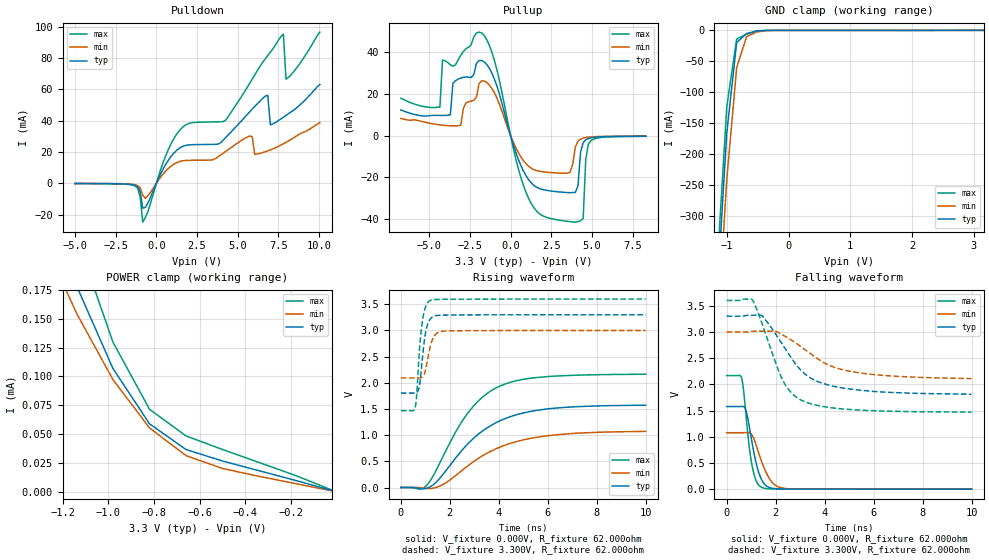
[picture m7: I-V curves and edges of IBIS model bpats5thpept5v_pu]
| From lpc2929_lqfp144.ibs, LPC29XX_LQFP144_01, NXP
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| |   Rev 0.20 IBIS Model Design Automation Generation   |
| |   N O N - S I L I C O N   C O R R E L A T E D   |
| |   This IBIS [Model] is pre-Beta tactical support   |
| |  Note: this IBIS [Model] contains clamp curves generated   |
| |   through simulation which should not be relied upon   |
| Pccmos14 hliolib_nlm 4.0.1
|   0.18 um 3.3V pad library
|   six level metal
|   dual oxide
|   single threshold voltage
|   nominal line mixed supply
|   parasitic extracted netlists
| Process block c14
| bpats5thpept5v
|   Bidirectional Pad 3v3
|   3state Output
|   Plain Input
|   5ns Slew Rate control
|   CMOS
|   Programmable between
|   - (p1=0, p2=1) plain input
|   - (p1=0, p2=0) with Pull Up
|   - (p1=1, p2=1) with Pull Down
|   - (p1=1, p2=0) with Repeater
|   Characterized at Core 1.8V and I/O 3.3V
| Pull Up Mode (p1=0, p2=0)
[Model]   bpats5thpept5v_pu | of bpats5thpept5v
Model_type   I/O
Polarity   Non-Inverting
Enable   Active-Low
|  Reciever Thresholds
Vinl   = 0.99V
Vinh   = 2.31V
| AC Test Load Conditions
Vref   = 0
Cref   = 1.2e-11
Rref   = 1000000000
Vmeas   = 1.65
| [Process Range]   typical   min   max
| C_comp edge width   400.000ps   400.000ps   400.000ps
| C_comp Tstrobe   40.000fs   40.000fs   40.000fs
C_comp   2.536pF   2.398pF   2.677pF
[Temperature Range]   25   125   -40
[Voltage Range]   3.30V   3.00V   3.60V
[GND Clamp Reference]   0.00V   0.00V   0.00V
[Pulldown Reference]   0.00V   0.00V   0.00V
[POWER Clamp Reference]   3.30V   3.00V   3.60V
[Pullup Reference]   3.30V   3.00V   3.60V
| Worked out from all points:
|   slope of the pulldown table from 0 to 0.495 V, typ, clamps not added: 46.5 ohm
|   slope of the pullup table from 0 to 0.495 V, typ, clamps not added: 41.9 ohm
|   GND clamp passes 1 mA (typ) near -0.48 V on its own axis
|   POWER clamp passes 1 mA (typ) near -2.29 V on its own axis
|   rising waveform, V_fixture 0.000V, R_fixture 62.000ohm: 20-80 % time 2.14ns typ, 2.37ns min, 1.8ns max; typ from 0.001 V to 1.57 V
|   falling waveform, V_fixture 0.000V, R_fixture 62.000ohm: 20-80 % time 411ps typ, 539ps min, 320ps max; typ from 1.58 V to 0.001 V
|   rising waveform, V_fixture 3.300V, R_fixture 62.000ohm: 20-80 % time 224ps typ, 260ps min, 214ps max; typ from 1.8 V to 3.3 V
|   falling waveform, V_fixture 3.300V, R_fixture 62.000ohm: 20-80 % time 1.53ns typ, 1.95ns min, 1.1ns max; typ from 3.3 V to 1.81 V
[GND Clamp]
| ref voltage   0.00V   0.00V   0.00V
|   Voltage   I(typ)   I(min)   I(max)
-5V       -7.933A    -7.953A    -7.929A
-1.16V    -429.6mA   -501mA     -389.4mA
-1V       -166.1mA   -240.8mA   -123.1mA
-840mV    -19.83mA   -60.19mA   -14.19mA
-680mV    -5.242mA   -10.3mA    -6.178mA
-520mV    -1.331mA   -2.714mA   -864.2uA
-200mV    -50.25uA   -41.81uA   -77.56uA
3.16V     -7.353uA   6.327uA    -29.63uA
[Power Clamp]   | Vtable = Vcc - Vpad
| ref voltage   3.30V   3.00V   3.60V
|   Voltage   I(typ)   I(min)   I(max)
-6.74V    8.239mA    4.142mA    14.64mA
-1.3V     267.9uA    224.8uA    334.3uA
-1.14V    178.7uA    154.9uA    220.9uA
-980mV    106.8uA    97.21uA    129.7uA
-820mV    58.96uA    55.39uA    71.57uA
-660mV    36.65uA    31.38uA    48.44uA
-500mV    26.73uA    20.24uA    36.7uA
-180mV    9.891uA    7.111uA    14.19uA
-20mV     1.102uA    817.7nA    1.531uA
[Pulldown]
| ref voltage   0.00V   0.00V   0.00V
|   Voltage   I(typ)   I(min)   I(max)
-5V       -187.5uA   -145.8uA   -211.8uA
-1.32V    -1.32mA    -939.5uA   -1.723mA
-840mV    -15.95mA   -7.735mA   -24.89mA
1.56V     23.24mA    14.25mA    35.29mA
4.28V     29.46mA    20.48mA    40.61mA
5.72V     45.48mA    30.13mA    63.63mA
6.84V     56.23mA    20.64mA    81.58mA
7V        37.28mA    21.27mA    83.66mA
7.8V      42.14mA    25.2mA     95.19mA
7.96V     43.32mA    26.11mA    66.52mA
8.12V     44.49mA    27.07mA    67.59mA
10.04V    63.09mA    38.66mA    96.53mA
[Pullup]   | Vtable = Vcc - Vpad
| ref voltage   3.30V   3.00V   3.60V
|   Voltage   I(typ)   I(min)   I(max)
-6.74V    12.27mA    8.208mA    17.93mA
-4.34V    9.688mA    5.132mA    13.69mA
-4.18V    9.676mA    4.983mA    36.31mA
-3.06V    27.66mA    4.956mA    38.56mA
-1.78V    36.09mA    26.29mA    49.34mA
940mV     -19.18mA   -13.46mA   -27.14mA
3.02V     -27.13mA   -18.05mA   -40.73mA
3.98V     -27.37mA   -5.511mA   -41.66mA
4.46V     -3.361mA   -1.235mA   -39.89mA
4.62V     -2.02mA    -961.6uA   -11.27mA
4.94V     -1.105mA   -662.3uA   -2.418mA
8.3V      -310.5uA   -276.1uA   -365.1uA
[Ramp]
R_load   = 62.000ohm
|   dV/dt(typ)   dV/dt(min)   dV/dt(max)
dV/dt_r   721.276mV/2.205ns   483.044mV/2.365ns   1.050V/2.040ns
dV/dt_f   673.548mV/1.570ns   397.074mV/1.940ns   1.036V/1.245ns
[Rising Waveform]  | cubic spline decimation from 2001 points
V_fixture   = 0.000V
R_fixture   = 62.000ohm
|   Time   V(typ)   V(min)   V(max)
0s        1.219mV    1.008mV    1.479mV
765ps     -15.82mV   -2.159mV   -31.04mV
1.06ns    -13.88mV   -16.43mV   44.85mV
1.715ns   248mV      56.81mV    587.1mV
2.695ns   814.7mV    399.6mV    1.397V
3.235ns   1.045V     578mV      1.685V
3.985ns   1.261V     760.1mV    1.926V
4.8ns     1.401V     886.9mV    2.049V
5.97ns    1.501V     987.6mV    2.118V
10ns      1.572V     1.072V     2.164V
[Falling Waveform]  | cubic spline decimation from 2001 points
V_fixture   = 0.000V
R_fixture   = 62.000ohm
|   Time   V(typ)   V(min)   V(max)
0s        1.577V     1.078V     2.168V
605ps     1.578V     1.078V     2.128V
680ps     1.578V     1.078V     1.924V
790ps     1.499V     1.079V     1.41V
1.025ns   920.6mV    1.039V     480.1mV
1.21ns    485.9mV    831.8mV    153mV
1.415ns   193.6mV    545.1mV    38.94mV
1.845ns   19.81mV    137.4mV    6.125mV
2.33ns    4.655mV    18.77mV    3.371mV
10ns      1.272mV    1.133mV    1.504mV
[Rising Waveform]  | cubic spline decimation from 2001 points
V_fixture   = 3.300V
V_fixture_min = 3.000V
V_fixture_max = 3.600V
R_fixture   = 62.000ohm
|   Time   V(typ)   V(min)   V(max)
0s        1.804V     2.094V     1.467V
585ps     1.804V     2.094V     1.535V
640ps     1.811V     2.094V     1.722V
745ps     1.908V     2.094V     2.524V
880ps     2.466V     2.115V     3.176V
1.01ns    2.96V      2.249V     3.45V
1.2ns     3.219V     2.693V     3.573V
1.425ns   3.282V     2.93V      3.592V
1.755ns   3.293V     2.987V     3.596V
10ns      3.3V       3V         3.6V
[Falling Waveform]  | cubic spline decimation from 2001 points
V_fixture   = 3.300V
V_fixture_min = 3.000V
V_fixture_max = 3.600V
R_fixture   = 62.000ohm
|   Time   V(typ)   V(min)   V(max)
0s        3.3V       3V         3.6V
1.04ns    3.32V      3.009V     3.616V
1.45ns    3.304V     3.014V     3.152V
2.045ns   2.93V      3.004V     2.354V
2.325ns   2.728V     2.933V     2.048V
2.68ns    2.477V     2.833V     1.821V
3.07ns    2.251V     2.706V     1.693V
3.76ns    2.046V     2.474V     1.593V
4.99ns    1.914V     2.253V     1.522V
10ns      1.812V     2.11V      1.471V
